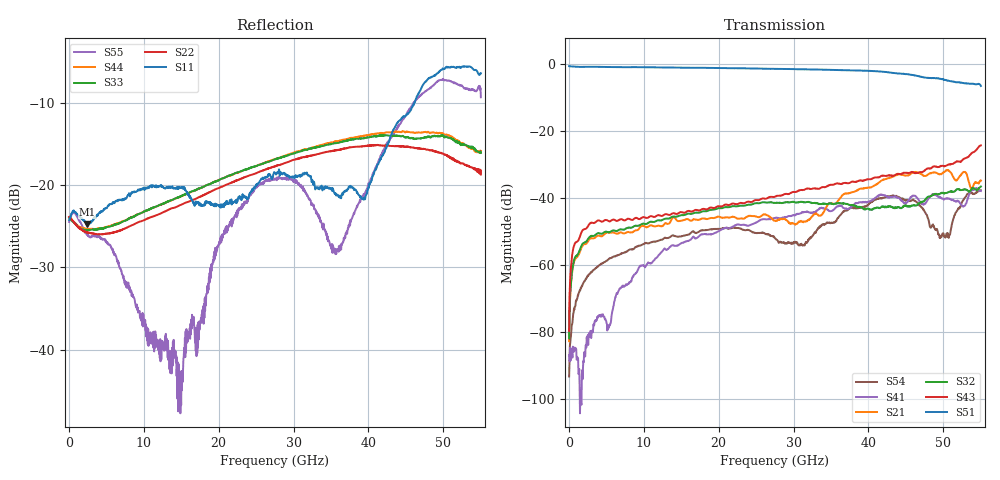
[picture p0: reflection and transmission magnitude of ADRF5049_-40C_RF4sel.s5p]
! Device  : ADRF5049
! Description: Silicon SP4T Switch Non-Reflective
! Frequency:  9kHz -  45 GHz
! Ports:
!  RFC = Port 1
!  RF1 = Port 2
!  RF2 = Port 3
!	 RF3 = Port 4
!  RF4 = Port 5
! VSS  =  +3.30 Volts
! VDD  =  -3.30 Volts
! EN  =  0.00 Volts
! LS  =  0.00 Volts
! V1  =  3.30 Volts
! V2  =  3.30 Volts
! Data:  Data was collected using an calibrated 4 port network analyzer.
! Notes: Analog Devices supplies this data as a sample of measured data
!  for this product.  Your particular data for this product may vary.
!  Data was taken at -40 degrees C.
!  Analog Devices reserves the right to change this data at anytime.
# ghz S db R 50
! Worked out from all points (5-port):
!   1100 points, 50 MHz to 55 GHz, reference 50 ohm
!   strongest paths, dB at 50 MHz, 13.8 GHz, 27.55 GHz, 41.3 GHz, 55 GHz:
!     S51: -0.6, -1.0, -1.4, -2.1, -6.5
!     S43: -79.6, -44.6, -39.5, -33.8, -24.2
!     S32: -81.9, -45.5, -41.4, -42.9, -36.5
!     S21: -82.7, -46.0, -46.7, -35.5, -34.7
!     S41: -86.8, -54.1, -45.9, -39.2, -37.8
!     S54: -93.2, -51.2, -51.9, -40.0, -37.6
!   lowest |S11| = -24.8 dB at 2.45 GHz (marker M1), VSWR 1.12, Z = 54.9 - j3.59 ohm
!   |S11| at or under -10 dB: start of sweep to 46.14 GHz
